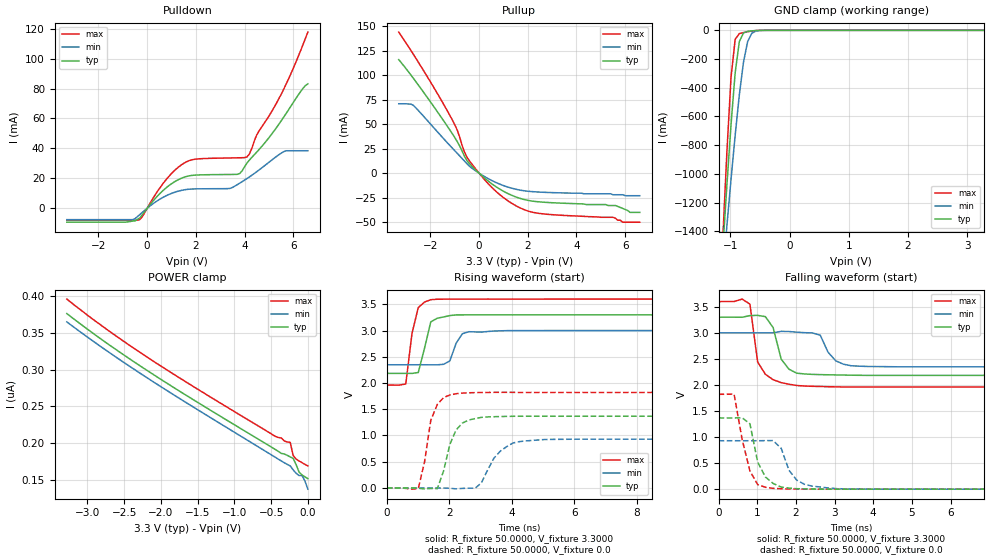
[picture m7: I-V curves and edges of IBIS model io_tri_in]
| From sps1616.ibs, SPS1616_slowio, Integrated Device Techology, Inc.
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|   Model io_tri_in
[Model]  io_tri_in
Model_type I/O
Polarity   Non-Inverting
Enable   Active-Low
Vinl =   0.8000V
Vinh =   2.0000V
Vmeas =  1.6500V
Cref =   50.0000pF
Rref =   1.0000M
Vref =   0.0V
C_comp   2.4706pF   2.4445pF   2.5092pF
[Temperature Range]   25.0000   0.1250k   -40.0000
[Voltage Range]   3.3000V   3.0000V   3.6000V
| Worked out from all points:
|   slope of the pulldown table from 0 to 0.495 V, typ, clamps not added: 52.7 ohm
|   slope of the pullup table from 0 to 0.495 V, typ, clamps not added: 47.9 ohm
|   GND clamp passes 1 mA (typ) near -0.54 V on its own axis
|   rising waveform, R_fixture 50.0000, V_fixture 3.3000: 20-80 % time 275ps typ, 289ps min, 269ps max; typ from 2.18 V to 3.3 V
|   rising waveform, R_fixture 50.0000, V_fixture 0.0: 20-80 % time 422ps typ, 631ps min, 367ps max; typ from 0 V to 1.37 V
|   falling waveform, R_fixture 50.0000, V_fixture 3.3000: 20-80 % time 292ps typ, 329ps min, 278ps max; typ from 3.3 V to 2.18 V
|   falling waveform, R_fixture 50.0000, V_fixture 0.0: 20-80 % time 329ps typ, 369ps min, 317ps max; typ from 1.37 V to 0 V
[Pulldown]
|Voltage   I(typ)   I(min)   I(max)
-3.3V     -9.3mA     -7.608mA   -8mA
-600mV    -8.526mA   -7.608mA   -8mA
-300mV    -6.39mA    -4.161mA   -7.475mA
700mV     12.56mA    7.713mA    17.54mA
1.5V      20.65mA    12.25mA    29.99mA
2V        22.18mA    12.95mA    32.85mA
3.4V      22.57mA    13.27mA    33.61mA
3.7V      22.68mA    15.77mA    33.7mA
4.1V      30.26mA    19.85mA    34.33mA
4.5V      37.53mA    24.43mA    49.05mA
5.6V      60.7mA     37.74mA    79.31mA
6.6V      83.15mA    38.43mA    117.7mA
[Pullup]
|Voltage   I(typ)   I(min)   I(max)
-3.3V     115.8mA    70.8mA     143.9mA
-2.7V     96.78mA    69.17mA    121.3mA
-1.1V     40.26mA    25.57mA    54.27mA
-900mV    32.28mA    20.29mA    44.08mA
-500mV    12.92mA    9.652mA    16.33mA
300mV     -6.55mA    -4.555mA   -8.729mA
1V        -18.43mA   -12.64mA   -24.91mA
1.7V      -25.83mA   -17.35mA   -35.57mA
2.3V      -28.84mA   -19.03mA   -40.38mA
5.6V      -33mA      -22mA      -46mA
5.9V      -36mA      -22mA      -50mA
6.6V      -40mA      -23mA      -50mA
[GND_clamp]
|Voltage   I(typ)   I(min)   I(max)
-3.3V     -16.98A    -12.79A    -23.09A
-1.13V    -1.531A    -1.696A    -1.457A
-1.06V    -1.079A    -1.362A    -847.9mA
-990mV    -656.4mA   -1.038A    -326.7mA
-920mV    -295.3mA   -730.3mA   -62.31mA
-850mV    -78.74mA   -450.3mA   -23.06mA
-780mV    -18.3mA    -223.2mA   -15.3mA
-710mV    -7.609mA   -79.38mA   -9.558mA
-640mV    -3.769mA   -20.78mA   -4.977mA
-570mV    -1.468mA   -4.666mA   -1.82mA
-360mV    -4.147uA   -27.64uA   -2.128uA
3.28V     150.9nA    171.3nA    151.2nA
[POWER_clamp]
|Voltage   I(typ)   I(min)   I(max)
-3.28V    376.1nA    364.8nA    395.8nA
-2.68V    332nA      321.7nA    350.6nA
-2V       286.8nA    276.8nA    304.8nA
-440mV    191.4nA    180.8nA    209.2nA
-360mV    186.2nA    175.9nA    207.2nA
-320mV    185.4nA    173.5nA    203nA
-240mV    181.5nA    169.3nA    201.2nA
-200mV    179.4nA    163.9nA    183.3nA
-120mV    160.9nA    156.2nA    176nA
-80mV     157nA      156.2nA    173.7nA
-40mV     154.4nA    148.8nA    171.4nA
0V        152nA      137.7nA    169.2nA
[Ramp]
| variable   typ   min   max
dV/dt_r  0.8202/0.4218n   0.5576/0.6213n   1.0926/0.3620n
dV/dt_f  0.6696/0.2824n   0.3912/0.3290n   0.9834/0.2779n
R_load = 50.0000
[Rising Waveform]
R_fixture= 50.0000
V_fixture= 3.3000
V_fixture_min= 3.0000
V_fixture_max= 3.6000
L_fixture= 0.0H
C_fixture= 0.0F
|time   V(typ)   V(min)   V(max)
0s        2.184V     2.348V     1.961V
610ps     2.184V     2.348V     1.982V
810ps     2.183V     2.348V     2.948V
1.01ns    2.2V       2.348V     3.438V
1.41ns    3.166V     2.347V     3.588V
2.02ns    3.285V     2.421V     3.599V
2.22ns    3.298V     2.758V     3.599V
2.42ns    3.298V     2.939V     3.599V
2.63ns    3.299V     2.978V     3.599V
20ns      3.3V       3V         3.6V
[Rising Waveform]
R_fixture= 50.0000
V_fixture= 0.0
V_fixture_min= 0.0
V_fixture_max= 0.0
L_fixture= 0.0H
C_fixture= 0.0F
|time   V(typ)   V(min)   V(max)
0s        2.794uV    3.322uV    2.602uV
1.01ns    -4.184mV   11.97uV    -12.39mV
1.21ns    -18.99mV   17.03uV    496.1mV
1.41ns    -9.484mV   65.24uV    1.29V
1.62ns    -12.69mV   -75.33uV   1.593V
2.22ns    1.106V     -17.26mV   1.796V
2.83ns    1.323V     -5.163mV   1.817V
3.64ns    1.361V     705.2mV    1.822V
4.44ns    1.367V     896.7mV    1.821V
20ns      1.367V     929.4mV    1.821V
[Falling Waveform]
R_fixture= 50.0000
V_fixture= 3.3000
V_fixture_min= 3.0000
V_fixture_max= 3.6000
L_fixture= 0.0H
C_fixture= 0.0F
|time   V(typ)   V(min)   V(max)
0s        3.3V       3V         3.6V
810ps     3.331V     3V         3.551V
1.01ns    3.335V     3V         2.44V
1.21ns    3.311V     2.999V     2.204V
1.41ns    3.101V     3V         2.101V
1.62ns    2.494V     3.028V     2.044V
2.02ns    2.226V     3.013V     1.989V
2.63ns    2.198V     2.955V     1.97V
3.64ns    2.185V     2.36V      1.961V
20ns      2.184V     2.348V     1.961V
[Falling Waveform]
R_fixture= 50.0000
V_fixture= 0.0
V_fixture_min= 0.0
V_fixture_max= 0.0
L_fixture= 0.0H
C_fixture= 0.0F
|time   V(typ)   V(min)   V(max)
0s        1.367V     929.5mV    1.821V
400ps     1.367V     929.4mV    1.824V
610ps     1.369V     929.4mV    949.8mV
810ps     1.255V     929.4mV    350.4mV
1.01ns    521.3mV    929.4mV    88.52mV
1.41ns    109.5mV    932.8mV    15.12mV
1.62ns    39.54mV    782.1mV    7.935mV
2.02ns    8.92mV     174.1mV    1.204mV
3.03ns    116.4uV    11.8mV     119.6uV
20ns      -1.58uV    1.975uV    5.015uV
